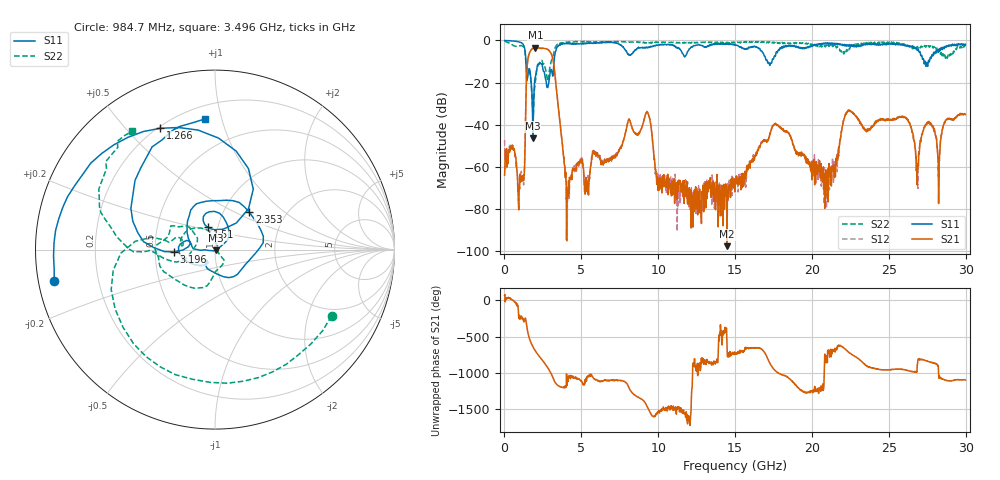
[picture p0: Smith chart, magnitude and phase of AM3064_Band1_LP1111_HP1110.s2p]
# Hz S DB R 50.0
!freq dBS11 angS11 dBS21 angS21 dBS12 angS12 dBS22 angS22
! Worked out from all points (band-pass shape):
!   1600 points, 10 MHz to 29.98 GHz, reference 50 ohm
!   highest |S21| = -3.44 dB at 2.016 GHz (marker M1); lowest = -97.7 dB at 14.48 GHz (marker M2)
!   |S21| within 3 dB of the highest: 1.605 GHz to 3.049 GHz (1.444 GHz wide, 62.1 % of centre)
!   lowest |S11| = -46.5 dB at 1.847 GHz (marker M3), VSWR 1.01, Z = 50.4 - j0.312 ohm
!   |S11| at or under -10 dB: 1.392 GHz to 3.226 GHz (1.834 GHz wide, 79.4 % of centre); 17.1 GHz to 17.4 GHz (299.4 MHz wide, 1.74 % of centre); 27.36 GHz to 27.57 GHz (207.8 MHz wide, 0.757 % of centre)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
!   |S22| runs from -36.2 to -0.2 dB; largest |S21 - S12| = 0.012
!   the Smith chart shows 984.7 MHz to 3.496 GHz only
!   S11 on the Smith chart (normalised r, x): 984.7 MHz: 0.05, -0.10; 1.266 GHz: 0.21, +0.63; 1.51 GHz: 0.89, +0.23; 2.353 GHz: 1.32, +0.60; 3.196 GHz: 0.63, -0.02; 3.496 GHz: 0.28, +0.89
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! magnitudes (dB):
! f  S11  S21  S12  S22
! 10 MHz  0.0  -64.0  -47.3  -0.2
! 984.7 MHz  -0.8  -70.6  -64.7  -2.5
! 1.266 GHz  -2.6  -63.8  -64.2  -3.5
! 1.51 GHz  -17.6  -9.7  -9.7  -14.9
! 1.847 GHz  -46.5  -3.9  -3.7  -34.7
! 2.016 GHz  -17.3  -3.4  -3.4  -19.4
! 2.353 GHz  -11.0  -3.8  -3.7  -9.9
! 3.196 GHz  -12.8  -10.8  -10.5  -6.4
! 3.496 GHz  -2.7  -31.4  -31.4  -1.9
! 4.096 GHz  -1.6  -74.4  -75.1  -0.9
! 5.015 GHz  -1.5  -56.5  -55.8  -0.6
! 9.288 GHz  -3.5  -34.2  -34.1  -1.3
! 10 GHz  -2.2  -69.8  -63.9  -0.9
! 14.48 GHz  -1.8  -97.7  -72.1  -1.0
! 15 GHz  -2.1  -66.6  -65.8  -1.2
! 17.59 GHz  -7.5  -39.9  -39.9  -1.0
! 19.99 GHz  -3.0  -66.1  -58.0  -1.8
! 21.38 GHz  -1.3  -59.4  -61.6  -2.7
! 22.35 GHz  -2.2  -33.3  -33.4  -4.3
! 25 GHz  -1.3  -37.8  -37.7  -1.1
! 26.85 GHz  -4.8  -68.7  -68.2  -2.9
! 29.98 GHz  -1.8  -35.2  -35.2  -2.8
